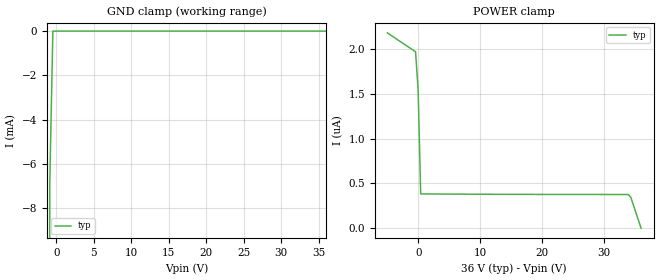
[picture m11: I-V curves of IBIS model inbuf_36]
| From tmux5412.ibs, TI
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| inbuf_36
[Model]   inbuf_36
Model_type   Input
Vinl = 0.8
Vinh = 1.3
|   typ   min   max
C_comp   1.598234e-12   NA   NA
[Voltage Range]   36   NA   NA
[Temperature Range]   27   NA   NA
[Power Clamp Reference]   36   NA   NA
[GND Clamp Reference]   0   NA   NA
[GND Clamp]
|   Voltage   I(typ)   I(min)   I(max)
-5V       -4.814A    NA         NA
-1.273V   -139.8mA   NA         NA
-858.6mV  -6.921mA   NA         NA
-444.4mV  -596.4nA   NA         NA
36V       1.153uA    NA         NA
[POWER Clamp]
|   Voltage   I(typ)   I(min)   I(max)
-5V       2.178uA    NA         NA
-444.4mV  1.968uA    NA         NA
-30.3mV   1.542uA    NA         NA
383.8mV   381.9nA    NA         NA
33.93V    375.4nA    NA         NA
34.34V    344nA      NA         NA
36V       -181.9pA   NA         NA
